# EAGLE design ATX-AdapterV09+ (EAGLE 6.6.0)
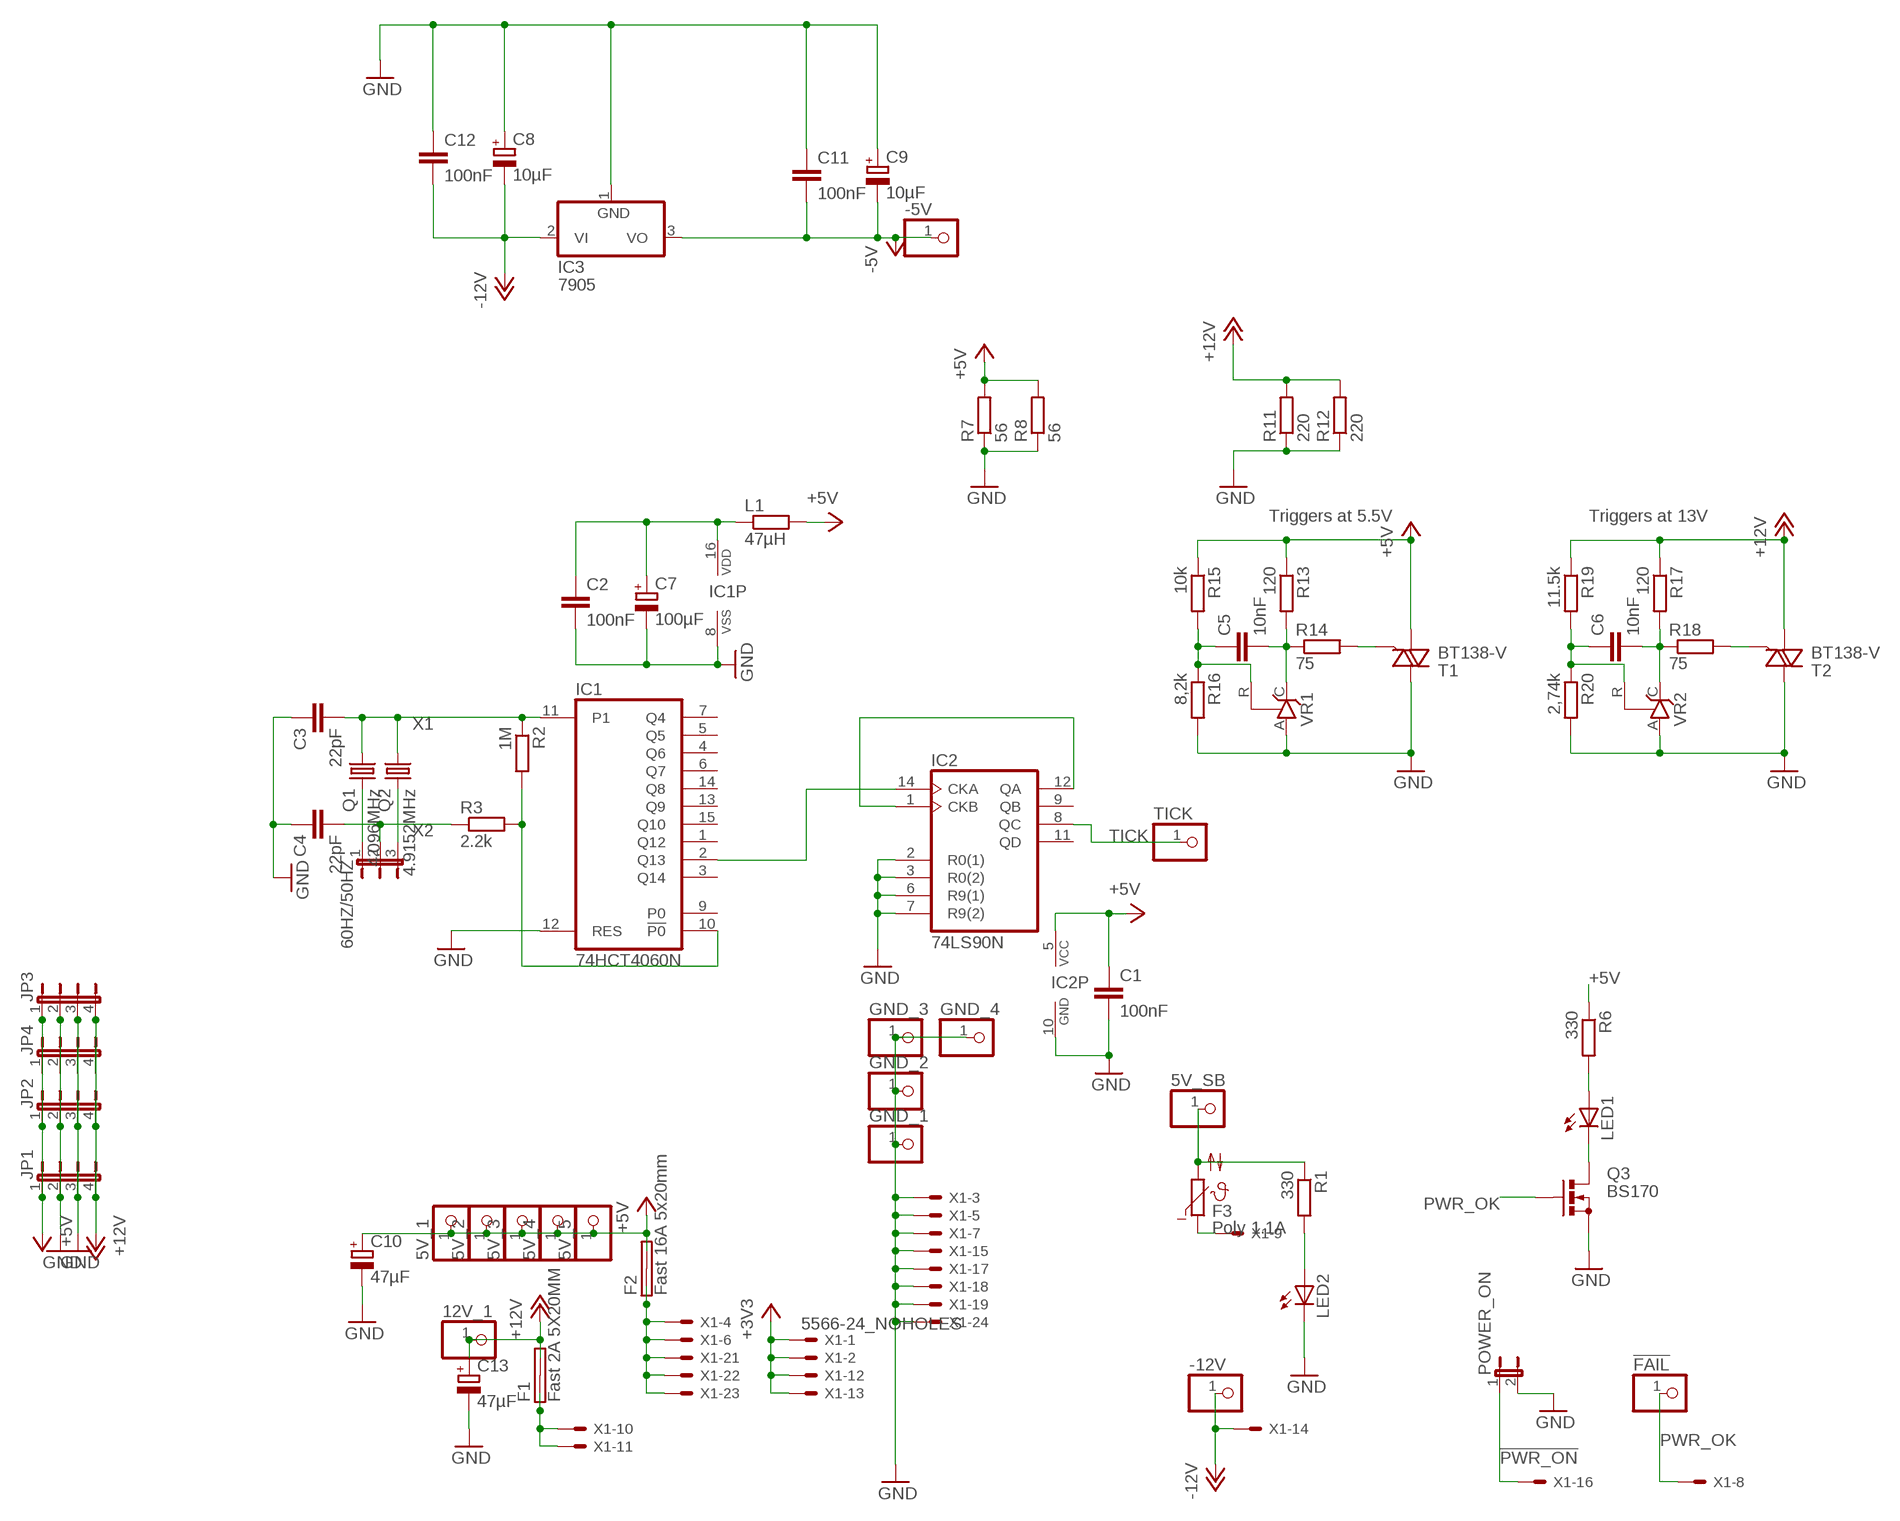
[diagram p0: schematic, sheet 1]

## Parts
5V_1  PINHD-1X1-LARGE  [1X01-LARGE]
5V_2  PINHD-1X1-LARGE  [1X01-LARGE]
5V_3  PINHD-1X1-LARGE  [1X01-LARGE]
5V_4  PINHD-1X1-LARGE  [1X01-LARGE]
5V_5  PINHD-1X1-LARGE  [1X01-LARGE]
5V_SB  PINHD-1X1_2.54  [1X01]
12V_1  PINHD-1X1-LARGE  [1X01-LARGE]
60HZ/50HZ  JP2E  [JP2]
!FAIL  PINHD-1X1_2.54  [1X01]
-5V  PINHD-1X1-LARGE  [1X01-LARGE]
-12V  PINHD-1X1-LARGE  [1X01-LARGE]
C1  100nF  C-EU025-025X050  [C025-025X050]
C2  100nF  C-EU025-025X050  [C025-025X050]
C3  22pF  C-EU025-025X050  [C025-025X050]
C4  22pF  C-EU025-025X050  [C025-025X050]
C5  10nF  C-EU025-025X050  [C025-025X050]
C6  10nF  C-EU025-025X050  [C025-025X050]
C7  100µF  CPOL-EUE5-5  [E5-5]
C8  10µF  CPOL-EUE5-5  [E5-5]
C9  10µF  CPOL-EUE5-5  [E5-5]
C10  47µF  CPOL-EUE5-5  [E5-5]
C11  100nF  C-EU025-025X050  [C025-025X050]
C12  100nF  C-EU025-025X050  [C025-025X050]
C13  47µF  CPOL-EUE5-5  [E5-5]
F1  Fast 2A 5X20MM  SHK20L  [SHK20L]
F2  Fast 16A 5x20mm  SHK20L  [SHK20L]
F3  Poly 1.1A  B57164  [B57164]
GND_1  PINHD-1X1-LARGE  [1X01-LARGE]
GND_2  PINHD-1X1-LARGE  [1X01-LARGE]
GND_3  PINHD-1X1-LARGE  [1X01-LARGE]
GND_4  PINHD-1X1-LARGE  [1X01-LARGE]
IC1  74HCT4060N  4060N  [DIL16]
IC2  74LS90N  [DIL14]
IC3  7905  7905TV  [TO220V]
JP1  JP4E  [JP4]
JP2  JP4E  [JP4]
JP3  JP4E  [JP4]
JP4  JP4E  [JP4]
L1  47µH  R-EU_0207/10  [0207/10]
LED1  LED3MM  [LED3MM]
LED2  LED3MM  [LED3MM]
POWER_ON  JP1E  [JP1]
Q1  4.096MHz  CRYSTALHC49S  [HC49/S]
Q2  4.9152MHz  CRYSTALHC49S  [HC49/S]
Q3  BS170  [SOT54E]
R1  330  R-EU_0204/7  [0204/7]
R2  1M  R-EU_0204/7  [0204/7]
R3  2.2k  R-EU_0204/7  [0204/7]
R6  330  R-EU_0204/7  [0204/7]
R7  56  R-EU_0414/15  [0414/15]
R8  56  R-EU_0414/15  [0414/15]
R11  220  R-EU_0414/15  [0414/15]
R12  220  R-EU_0414/15  [0414/15]
R13  120  R-EU_0204/7  [0204/7]
R14  75  R-EU_0204/7  [0204/7]
R15  10k  R-EU_0204/7  [0204/7]
R16  8,2k  R-EU_0204/7  [0204/7]
R17  120  R-EU_0204/7  [0204/7]
R18  75  R-EU_0204/7  [0204/7]
R19  11.5k  R-EU_0204/7  [0204/7]
R20  2,74k  R-EU_0204/7  [0204/7]
T1  BT138-V  [TO220BV]
T2  BT138-V  [TO220BV]
TICK  PINHD-1X1-LARGE  [1X01-LARGE]
VR1  TL431CLP  [TO92-CLP]
VR2  TL431CLP  [TO92-CLP]
X1  5566-24_NOHOLES  [5566-24B]

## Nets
5V_ATX: F2.1A F2.1B X1.4 X1.6 X1.21 X1.22 X1.23
5V_SB: F3.1 X1.9
!PWR_ON: POWER_ON.1 X1.16
+3V3: X1.1 X1.2 X1.12 X1.13
+5V: 5V_1.1 5V_2.1 5V_3.1 5V_4.1 5V_5.1 C1.1 C10.+ F2.2A F2.2B IC2.5(VCC) JP1.1 JP2.1 JP3.1 JP4.1 L1.2 R6.1 R7.2 R8.2 R13.1 R15.1 T1.T1(A1)
+12V: 12V_1.1 C13.+ F1.2A F1.2B JP1.4 JP2.4 JP3.4 JP4.4 R11.2 R12.2 R17.1 R19.1 T2.T1(A1)
-5V: -5V.1 C9.- C11.2 IC3.3(VO)
-12V: -12V.1 C8.- C12.2 IC3.2(VI) X1.14
GND: C1.2 C2.2 C3.1 C4.1 C7.- C8.+ C9.+ C10.- C11.1 C12.1 C13.- GND_1.1 GND_2.1 GND_3.1 GND_4.1 IC1.8(VSS) IC1.12(RES) IC2.2(R0(1)) IC2.3(R0(2)) IC2.6(R9(1)) IC2.7(R9(2)) IC2.10(GND) IC3.1(GND) JP1.2 JP1.3 JP2.2 JP2.3 JP3.2 JP3.3 JP4.2 JP4.3 LED2.K(C) POWER_ON.2 Q3.S R7.1 R8.1 R11.1 R12.1 R16.2 R20.2 T1.T2(A2) T2.T2(A2) VR1.A VR2.A X1.3 X1.5 X1.7 X1.15 X1.17 X1.18 X1.19 X1.24
N$1: LED2.A R1.2
N$2: IC1.2(Q13) IC2.14(CKA)
N$4: 60HZ/50HZ.1 Q1.2
N$5: 60HZ/50HZ.3 Q2.2
N$6: 5V_SB.1 F3.2 R1.1
N$7: IC1.10(!P0) R2.2 R3.2
N$8: IC2.1(CKB) IC2.12(QA)
N$10: LED1.A R6.2
N$11: F1.1A F1.1B X1.10 X1.11
N$12: C2.1 C7.+ IC1.16(VDD) L1.1
N$13: R14.2 T1.G
N$14: C5.2 R13.2 R14.1 VR1.C
N$15: C5.1 R15.2 R16.1 VR1.R
N$17: R18.2 T2.G
N$18: C6.2 R17.2 R18.1 VR2.C
N$19: C6.1 R19.2 R20.1 VR2.R
N$20: LED1.K(C) Q3.D
PWR_OK: !FAIL.1 Q3.G X1.8
TICK: IC2.8(QC) TICK.1
X1: C3.2 IC1.11(P1) Q1.1 Q2.1 R2.1
X2: 60HZ/50HZ.2 C4.2 R3.1
Unconnected: IC1.1(Q12) IC1.3(Q14) IC1.4(Q6) IC1.5(Q5) IC1.6(Q7) IC1.7(Q4) IC1.9(P0) IC1.13(Q9) IC1.14(Q8) IC1.15(Q10) IC2.9(QB) IC2.11(QD) X1.20

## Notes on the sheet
- Triggers at 5.5V | Triggers at 13V

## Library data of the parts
5V_1-5V_5 5V_SB 12V_1 !FAIL -5V -12V GND_1-GND_4 TICK = pinhead:PINHD-1X1: PIN HEADER
60HZ/50HZ = jumper:JP2E: JUMPER
C1-C6 C11 C12 = rcl:C-EU: CAPACITOR, European symbol
C7-C10 C13 = rcl:CPOL-EU: POLARIZED CAPACITOR, European symbol
F1 F2 = fuse:SHK20L: FUSE HOLDER 5 x 20 mm, SH contact, SHH1 Schukat, E1073 Buerklin; OC_FARNELL: unknown; OC_NEWARK: unknown
F3 = ptc-ntc:B57164: SIEMENS NTC; MPN: B57164K474K52; OC_FARNELL: 9753451; OC_NEWARK: 29M3118
IC1 = 40xx:4060: 14-stage binary/ripple COUNTER
IC2 = 74xx-eu:74*90: Decade, divide by twelve and binary COUNTER
IC3 = linear:79*: Negative VOLTAGE REGULATOR
JP1-JP4 = jumper:JP4E: JUMPER
L1 R1-R3 R6 R13-R20 = rcl:R-EU_: RESISTOR, European symbol
LED1 LED2 = led:LED: LED
POWER_ON = jumper:JP1E: JUMPER
Q1 Q2 = crystal:CRYSTAL: CRYSTAL; OC_FARNELL: 1667008; OC_NEWARK: unknown
Q3 = transistor-small-signal:BS170: N-CHANNEL MOS FET
R7 R8 R11 R12 = resistor:R-EU_: RESISTOR, European symbol
T1 T2 = triac:BT138: TRIAC Source: http://www.semiconductors.philips.com BT138_SERIES_2.pdf
VR1 VR2 = v-reg:TL431CLP: VOLTAGE REGULATOR
X1 = con-molex:5566-24: Mini FIT connector 24 pol Source: http://www.molex.com

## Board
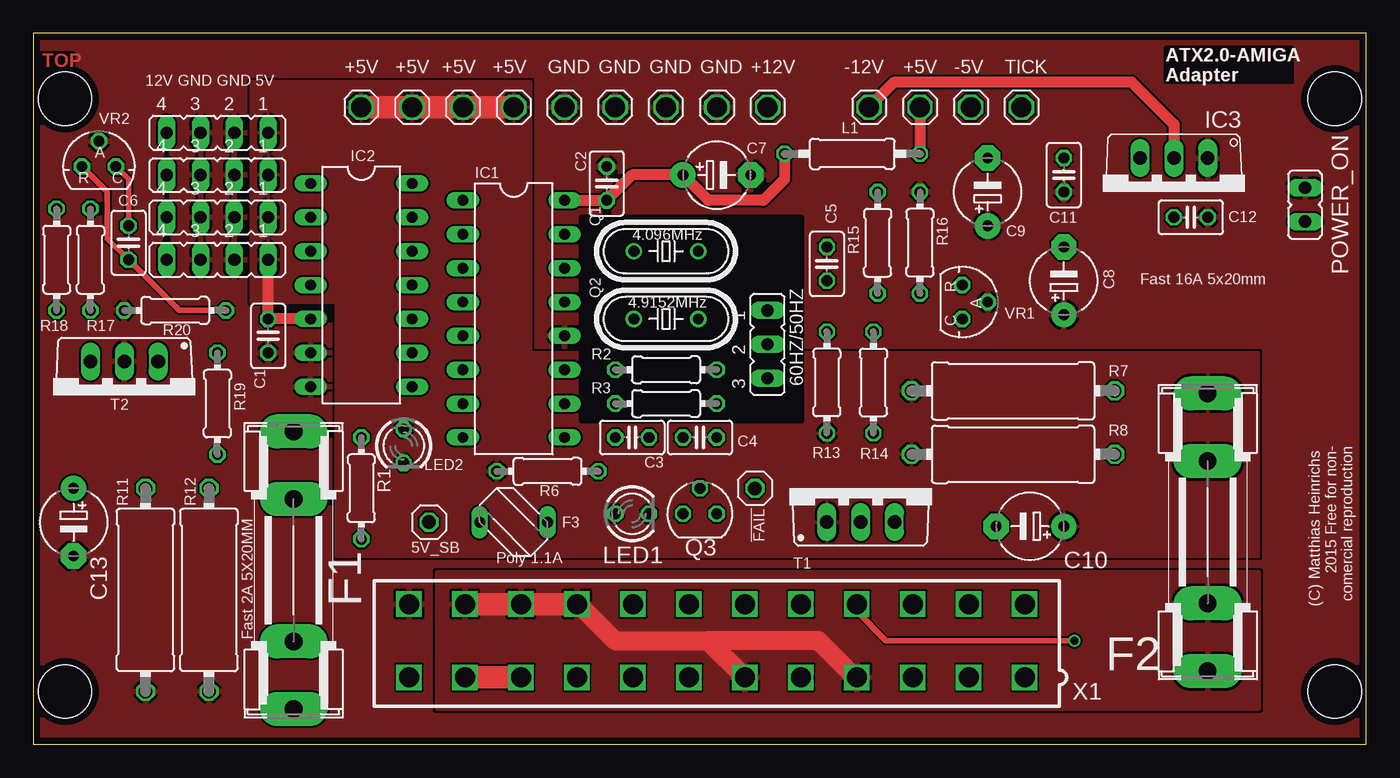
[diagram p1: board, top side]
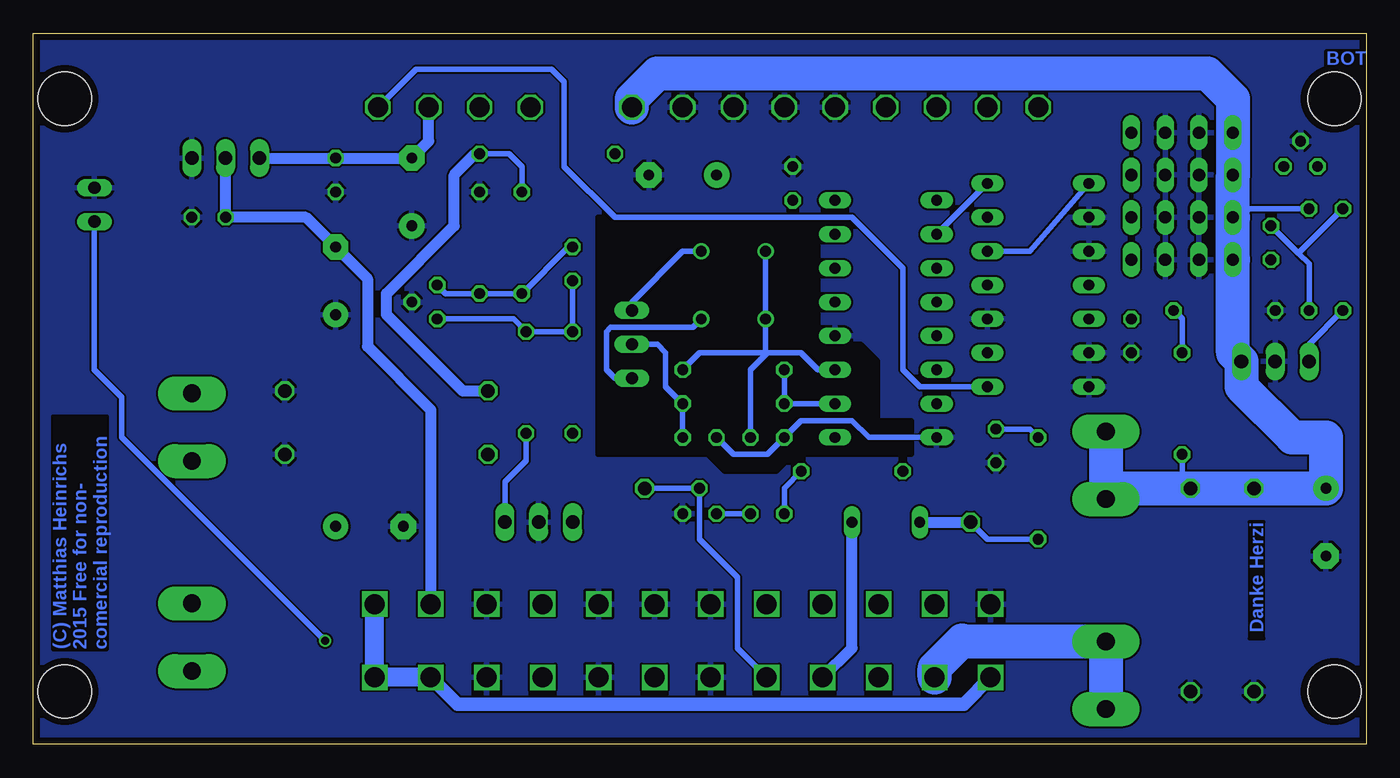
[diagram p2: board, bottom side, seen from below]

Size 99.99 x 53.33 mm. Coordinates in mm from the lower left corner, seen from the top.
Outline: 0,0 99.99,0 99.99,53.33 0,53.33 0,0
Copper layers (1*16): Top 0.035mm / dielectric 1.5mm / Bottom 0.035mm
Design rules "Eagle-DRU - 1203 - LeitOn - 01 and 02 layers": minimum track width 6mil, minimum drill 0.3mm, track to track 6mil, track to pad 6mil, pad to pad 6mil, via to via 6mil, smd to smd 6mil, copper to edge 20mil, drill to drill 10mil, minimum pad ring 8mil, minimum via ring 6mil, stop-mask expansion 3mil, vias tented up to drill 0mil, thermal gap 8mil
Holes 4 mm at 2.38,3.97 97.63,3.97 97.63,48.42 2.38,48.42

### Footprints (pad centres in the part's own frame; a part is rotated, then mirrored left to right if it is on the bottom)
1X01-LARGE = drill 1.5 octagon: 1 0,0
1X01 = drill 1.016 octagon: 1 0,0
JP2 = drill 0.914 long: 1 -2.54,0; 2 0,0; 3 2.54,0
C025-025X050 = drill 0.813 octagon: 1 -1.27,0; 2 1.27,0
E5-5 = drill 0.813 pad 1.905: + -2.54,0 | drill 0.813 pad 1.905 octagon: - 2.54,0
SHK20L = drill 1.321 pad 2.54 long: 1A -10.414,0; 1B -5.334,0; 2A 10.414,0; 2B 5.334,0
B57164 = drill 0.813 long: 1 -2.54,0; 2 2.54,0
DIL16 = drill 0.813 long: 1 -8.89,-3.81; 2 -6.35,-3.81; 3 -3.81,-3.81; 4 -1.27,-3.81; 5 1.27,-3.81; 6 3.81,-3.81; 7 6.35,-3.81; 8 8.89,-3.81; 9 8.89,3.81; 10 6.35,3.81; 11 3.81,3.81; 12 1.27,3.81; 13 -1.27,3.81; 14 -3.81,3.81; 15 -6.35,3.81; 16 -8.89,3.81
DIL14 = drill 0.813 long: 1 -7.62,-3.81; 2 -5.08,-3.81; 3 -2.54,-3.81; 4 0,-3.81; 5 2.54,-3.81; 6 5.08,-3.81; 7 7.62,-3.81; 8 7.62,3.81; 9 5.08,3.81; 10 2.54,3.81; 11 0,3.81; 12 -2.54,3.81; 13 -5.08,3.81; 14 -7.62,3.81
TO220V = drill 1.016 long: 1 -2.54,-2.54; 2 0,-2.54; 3 2.54,-2.54
JP4 = drill 0.914 long: 1 -3.81,0; 2 -1.27,0; 3 1.27,0; 4 3.81,0
0207/10 = drill 0.813 octagon: 1 -5.08,0; 2 5.08,0
LED3MM = drill 0.813 octagon: A -1.27,0; K 1.27,0
JP1 = drill 0.914 long: 1 0,-1.27; 2 0,1.27
HC49/S = drill 0.813: 1 -2.413,0; 2 2.413,0
SOT54E = drill 0.813 octagon: D -1.27,0; G 0,1.905; S 1.27,0
0204/7 = drill 0.813 octagon: 1 -3.81,0; 2 3.81,0
0414/15 = drill 1.016 octagon: 1 -7.62,0; 2 7.62,0
TO220BV = drill 1.016 long: G 2.54,-2.54; T1 -2.54,-2.54; T2 0,-2.54
TO92-CLP = drill 0.813 octagon: A 0,1.905; C 1.27,0; R -1.27,0
5566-24B = drill 1.5 square: 1 23.1,-2.75; 2 18.9,-2.75; 3 14.7,-2.75; 4 10.5,-2.75; 5 6.3,-2.75; 6 2.1,-2.75; 7 -2.1,-2.75; 8 -6.3,-2.75; 9 -10.5,-2.75; 10 -14.7,-2.75; 11 -18.9,-2.75; 12 -23.1,-2.75; 13 23.1,2.75; 14 18.9,2.75; 15 14.7,2.75; 16 10.5,2.75; 17 6.3,2.75; 18 2.1,2.75; 19 -2.1,2.75; 20 -6.3,2.75; 21 -10.5,2.75; 22 -14.7,2.75; 23 -18.9,2.75; 24 -23.1,2.75

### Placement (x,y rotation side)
5V_1  24.61,47.78 0 top
5V_2  28.42,47.78 0 top
5V_3  32.23,47.78 0 top
5V_4  36.04,47.78 0 top
5V_5  66.52,47.78 0 top
5V_SB  29.69,16.67 0 top
12V_1  55.09,47.78 0 top
60HZ/50HZ  55.09,30 270 top
!FAIL  54.13,19.21 0 top
-5V  70.33,47.78 0 top
-12V  62.71,47.78 0 top
C1  17.62,30.64 270 top
C2  43.02,42.07 90 top
C3  44.93,23.02 0 top
C4  50.01,23.02 0 top
C5  59.53,36.04 270 top
C6  7.14,37.62 90 top
C7  51.28,42.7 0 top
C8  77.31,34.77 90 top
C9  71.6,41.43 90 top
C10  74.77,16.35 180 top
C11  77.31,42.7 90 top
C12  86.84,39.53 180 top
C13  3.02,16.67 270 top
F1  19.53,13.06 90 top
F2  88.11,15.92 90 top
F3  36.04,16.67 180 top
GND_1  39.85,47.78 180 top
GND_2  43.66,47.78 180 top
GND_3  47.47,47.78 180 top
GND_4  51.28,47.78 0 top
IC1  36.04,31.91 270 top
IC2  24.61,34.45 270 top
IC3  85.57,41.43 180 top
JP1  13.81,42.7 180 top
JP2  13.81,39.53 180 top
JP3  13.81,36.35 180 top
JP4  13.81,45.88 180 top
L1  61.44,44.29 0 top
LED1  44.93,17.3 0 top
LED2  27.78,22.38 270 top
POWER_ON  95.41,40.48 0 top
Q1  47.47,36.99 0 top
Q2  47.47,31.91 0 top
Q3  50.01,17.3 0 top
R1  24.61,19.21 90 top
R2  47.47,28.1 180 top
R3  47.47,25.56 180 top
R6  38.58,20.48 0 top
R7  73.5,26.51 180 top
R8  73.5,21.75 180 top
R11  8.41,11.59 90 top
R12  13.18,11.59 90 top
R13  59.53,27.15 90 top
R14  63.02,27.15 270 top
R15  63.34,37.62 270 top
R16  66.52,37.62 90 top
R17  4.29,36.35 270 top
R18  1.75,36.35 270 top
R19  13.81,25.56 90 top
R20  10.64,32.54 180 top
T1  62.07,19.21 0 top
T2  6.83,26.19 180 top
TICK  74.14,47.78 0 top
VR1  69.69,33.18 270 top
VR2  4.92,43.34 0 top
X1  51.28,7.78 0 top

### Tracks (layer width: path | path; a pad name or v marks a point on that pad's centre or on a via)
5V_ATX
  Top 1.422: X1.21 40.91,10.53 43.66,7.78 50.63,7.78 | 50.63,7.78 X1.6 | X1.4 61.65,5.03 58.9,7.78 50.63,7.78
  Top 1.676: X1.23 X1.22 X1.21
  pour Top: 30.32,12.86 91.92,12.86 91.92,2.7 30.32,2.7
5V_SB
  Bottom 0.813: X1.9 38.58,7.23 F3.1
!PWR_ON  (via drill 0.6)
  Top 0.406: X1.16 61.78,9.98 63.98,7.78 v78.11,7.78
  Bottom 0.406: v78.11,7.78 93.34,23.02 93.34,26.04 95.41,28.1 POWER_ON.1
+3V3
  Bottom 1.016: X1.2 68.16,3.02 30.19,3.02 X1.12
  Bottom 1.422: X1.13 X1.1 X1.2
+5V
  Top 0.813: IC2.5 C1.1 JP3.1 | 5V_5.1 L1.2
  Top 1.676: 5V_1.1 5V_2.1 5V_3.1 5V_4.1
  Bottom 0.406: R15.1 63.34,43.34 64.29,44.29 L1.2
  Bottom 0.813: L1.2 66.83,44.29 68.42,42.7 68.42,38.89 73.5,33.81 73.5,32.23 67.79,26.51 R7.2
  pour Top: 16.35,49.69 37.31,49.69 37.31,29.37 91.92,29.37 91.92,14.13 22.7,14.13 22.7,33.18 16.35,33.18
+12V
  Bottom 0.406: R19.1 13.81,19.84 R12.2 | R17.1 10,40.16
  Bottom 2.54: 12V_1.1 55.09,48.42 53.18,50.32 11.91,50.32 10,48.42 JP4.4 JP1.4 10,40.16 JP2.4 JP3.4 10,29.37 T2.T1 9.37,26.83 5.56,23.02 3.02,23.02 C13.+ R11.2 R12.2 19.53,19.21 F1.2B F1.2A
-5V
  Bottom 0.406: -5V.1 70.33,47.15
  Bottom 0.813: -5V.1 70.33,45.24 C9.- C11.2 IC3.3
-12V
  Top 0.813: -12V.1 64.61,49.69 82.39,49.69 85.57,46.51 IC3.2
  Bottom 0.813: X1.14 70.18,25.09 74.93,29.84 74.93,34.93 C8.- 79.53,39.53 C12.2 IC3.2
GND
  Bottom 0.406: C4.1 47.47,21.75 44.93,21.75 C3.1 42.39,24.29 38.58,24.29 37.31,23.02 IC1.8
  pour Bottom (rank 2): 0,0 100.01,0 100.01,53.34 0,53.34
  pour Top (rank 2): 0,0 100.01,0 100.01,53.34 0,53.34
N$1
  Bottom 0.406: LED2.A 25.24,23.65 R1.2
N$2
  Bottom 0.406: IC2.14 IC1.2
N$3
  cutout Bottom: 41.12,39.53 57.63,39.53 57.63,21.75 49.37,21.75 48.1,20.48 44.29,20.48 43.02,21.75 34.13,21.75 34.13,24.29 36.67,24.29 36.67,28.73 37.94,30 41.12,30
  cutout Top: 41.12,39.53 57.63,39.53 57.63,24.29 41.12,24.29
N$4
  Bottom 0.406: Q1.2 51.28,36.99 55.09,33.18 60HZ/50HZ.1
N$5
  Bottom 0.406: 60HZ/50HZ.3 56.36,27.46 56.99,28.1 56.99,30.96 56.67,31.27 50.51,31.27 Q2.2
N$6
  Bottom 0.406: 5V_SB.1 28.42,15.4 R1.1
  Bottom 0.813: F3.2 5V_SB.1
N$7
  Bottom 0.406: R2.2 R3.2 IC1.10
N$8
  Bottom 0.406: IC2.12 25.24,36.99 IC2.1
N$10
  Bottom 0.406: LED1.A 43.66,19.21 R6.2
N$11
  Top 1.676: X1.10 X1.11
  Bottom 2.54: X1.11 32.38,5.72 30.32,7.78 30.27,7.73 F1.1B F1.1A
N$12
  Top 0.813: IC1.16 C2.1 44.93,42.7 C7.+ 50.64,40.8 54.77,40.8 56.36,42.39 L1.1
N$13
  Bottom 0.406: T1.G 64.61,19.68 63.02,21.27 R14.2
N$14
  Bottom 0.406: C5.2 R13.2 R14.1 63.98,31.91 VR1.C
N$15
  Bottom 0.406: C5.1 59.85,37.31 R15.2 R16.1 69.06,33.81 VR1.R
N$17
  Bottom 0.406: R18.2 4.29,30 T2.G
N$18
  Top 0.406: C6.2 7.14,42.39 VR2.C
  Bottom 0.406: R17.2 4.29,36.04 5.08,36.83 | 5.08,36.83 C6.2 | R18.1 5.08,36.83
N$19
  Top 0.406: VR2.R 5.56,41.43 5.56,37.94 C6.1 10.95,32.54 R20.1
  Bottom 0.406: R20.1 13.81,31.91 R19.2
N$20
  Bottom 0.406: LED1.K Q3.D
PWR_OK
  Bottom 0.406: X1.8 47.15,7.2 47.15,12.54 50.01,15.4 Q3.G !FAIL.1
TICK
  Bottom 0.406: TICK.1 71.28,50.64 61.12,50.64 60.17,49.69 60.17,43.34 56.36,39.53 38.58,39.53 34.77,35.72 34.77,28.1 33.5,26.83 IC2.8
X1
  Bottom 0.406: Q1.1 Q2.1 45.05,29.5 44.93,29.37 | IC1.11 41.12,28.1 42.39,29.37 44.93,29.37 | 44.93,29.37 50.01,29.37 R2.1 | C3.2 46.2,28.1 44.93,29.37
X2
  Bottom 0.406: C4.2 R3.1 52.55,26.83 52.55,29.37 53.18,30 60HZ/50HZ.2

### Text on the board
Top: TOP | ATX2.0-AMIGA / Adapter
Bottom: BOT | Danke Herzi | (C) Matthias Heinrichs / 2015 Free for non- / comercial reproduction
tNames: +5V | +5V | +5V | +5V | GND | GND | GND | GND | +12V | -12V | +5V | -5V | TICK | 12V GND GND 5V | ATX2.0-AMIGA / Adapter | (C) Matthias Heinrichs / 2015 Free for non- / comercial reproduction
